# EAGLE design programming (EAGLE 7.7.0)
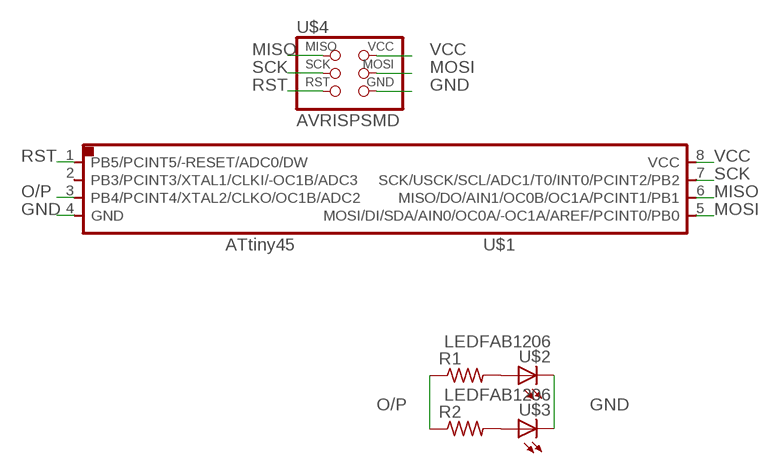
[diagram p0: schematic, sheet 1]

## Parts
R1  RES-US1206FAB  [R1206FAB]
R2  RES-US1206FAB  [R1206FAB]
U$1  ATTINY45SI  [SOIC8]
U$2  LEDFAB1206  [LED1206FAB]
U$3  LEDFAB1206  [LED1206FAB]
U$4  AVRISPSMD  [2X03SMD]

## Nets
GND: U$1.4(GND) U$2.2(C) U$3.2(C) U$4.6(GND)
MISO: U$1.6(MISO/DO/AIN1/OC0B/OC1A/PCINT1/PB1) U$4.1(MISO)
MOSI: U$1.5(MOSI/DI/SDA/AIN0/OC0A/-OC1A/AREF/PCINT0/PB0) U$4.4(MOSI)
N$3: R1.2 U$2.1(A)
N$4: R2.2 U$3.1(A)
O/P: R1.1 R2.1 U$1.3(PB4/PCINT4/XTAL2/CLKO/OC1B/ADC2)
RST: U$1.1(PB5/PCINT5/-RESET/ADC0/DW) U$4.5(RST)
SCK: U$1.7(SCK/USCK/SCL/ADC1/T0/INT0/PCINT2/PB2) U$4.3(SCK)
VCC: U$1.8(VCC) U$4.2(VCC)
Unconnected: U$1.2(PB3/PCINT3/XTAL1/CLKI/-OC1B/ADC3)

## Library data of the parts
R1 R2 = fab:RES-US: Resistor (US Symbol)
U$1 = fab:ATTINY45
U$2 U$3 = fab:LED: LED
U$4 = fab:AVRISP

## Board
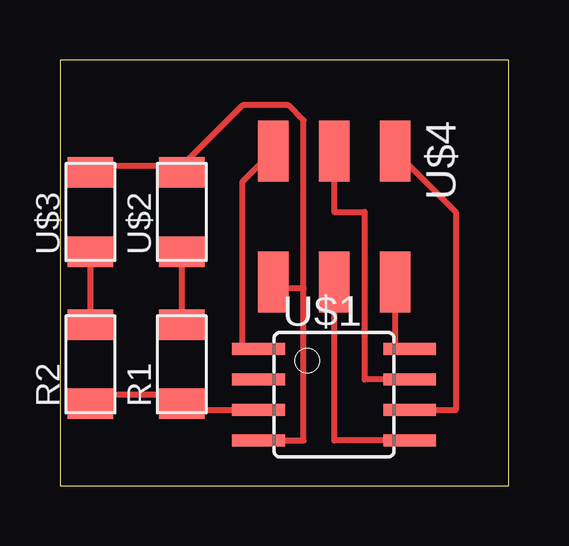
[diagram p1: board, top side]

Size 18.72 x 17.77 mm. Coordinates in mm from the lower left corner, seen from the top.
Outline: 0,0 18.72,0 18.72,17.77 0,17.77 0,0
Copper layers (1*16): Top 0.035mm / dielectric 1.5mm / Bottom 0.035mm
Design rules "default": minimum track width 10mil, minimum drill 24mil, track to track 8mil, track to pad 8mil, pad to pad 8mil, via to via 8mil, smd to smd 8mil, copper to edge 40mil, drill to drill 8mil, minimum pad ring 10mil, minimum via ring 8mil, stop-mask expansion 4mil, vias tented up to drill 0mil, thermal gap 10mil

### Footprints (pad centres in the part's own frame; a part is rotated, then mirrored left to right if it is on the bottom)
R1206FAB = smd 1.27 x 1.905: 1 -1.651,0; 2 1.651,0
SOIC8 = smd 0.5 x 2.2: 1 -1.905,-3.154; 2 -0.645,-3.154; 3 0.625,-3.154; 4 1.895,-3.154; 5 1.905,3.154; 6 0.635,3.154; 7 -0.635,3.154; 8 -1.905,3.154
LED1206FAB = smd 1.27 x 1.905: 1 -1.651,0; 2 1.651,0
2X03SMD = smd 2.54 x 1.27: 1 -2.54,2.54; 2 2.92,2.54; 3 -2.54,0; 4 2.92,0; 5 -2.54,-2.54; 6 2.92,-2.54

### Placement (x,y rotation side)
R1  5.08,5.08 90 top
R2  1.27,5.08 90 top
U$1  11.43,3.81 270 top
U$2  5.08,11.43 90 top
U$3  1.27,11.43 90 top
U$4  11.43,11.43 270 top

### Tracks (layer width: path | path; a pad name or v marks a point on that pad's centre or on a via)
GND
  Top 0.254: 5.08,13.34 1.27,13.34 U$3.2 | U$1.4 8.89,1.91 10.16,1.91 10.16,8.26 | U$4.6 8.89,8.26 10.16,8.26 | 5.08,13.34 7.62,15.88 9.53,15.88 10.16,15.24 10.16,8.26 | 5.08,13.34 U$2.2
MISO
  Top 0.254: U$4.1 16.51,11.43 16.51,3.17 U$1.6
MOSI
  Top 0.254: U$4.4 11.43,1.91 U$1.5
N$3
  Top 0.254: U$2.1 R1.2
N$4
  Top 0.254: U$3.1 R2.2
O/P
  Top 0.254: R2.1 1.27,3.81 5.08,3.81 R1.1 5.08,3.17 8.26,3.17 U$1.3
RST
  Top 0.254: U$4.5 7.62,12.7 7.62,5.71 U$1.1
SCK
  Top 0.254: U$1.7 12.7,4.45 12.7,11.43 11.43,11.43 U$4.3
VCC
  Top 0.254: U$4.2 13.97,5.71 U$1.8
